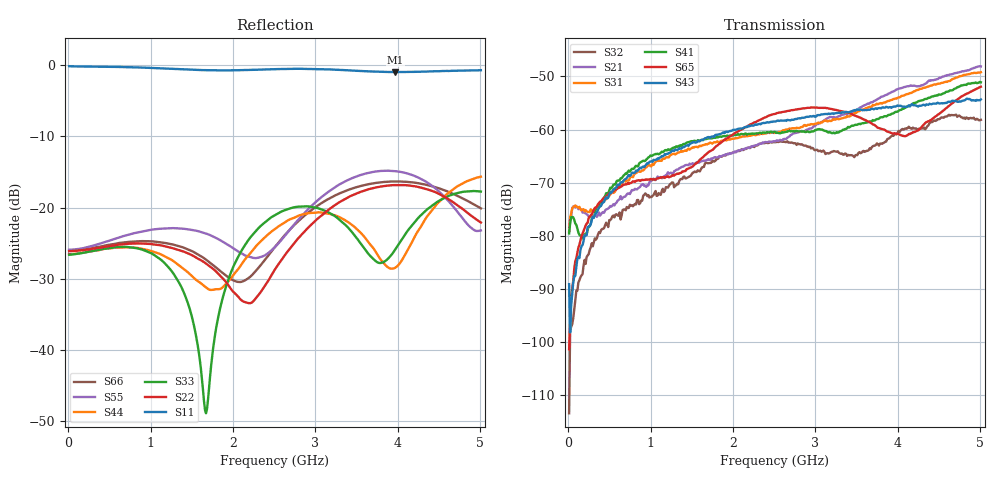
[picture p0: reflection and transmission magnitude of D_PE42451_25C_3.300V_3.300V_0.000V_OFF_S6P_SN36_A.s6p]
! Device ID: PE42451
! Serial: 36
! Insertion: A
! Temp: 25C
! VDD: 3.300
! Control_Hi: 100.000
! Control_Lo: 0.000
! Logic State: OFF
! Port 1: RFC
! Port 2: RF1
! Port 3: RF2
! Port 4: RF3
! Port 5: RF4
! Port 6: RF5
! V1 = 0.00
! V2 = 3.30
! V3 = 3.30
! V4 = 0.00
! IDD: 1.594190e-05
#  Hz  S  RI  R  50
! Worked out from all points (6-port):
!   401 points, 10 MHz to 5.01 GHz, reference 50 ohm
!   strongest paths, dB at 10 MHz, 1.26 GHz, 2.51 GHz, 3.76 GHz, 5.01 GHz:
!     S43: -89.1, -64.0, -58.5, -56.0, -54.3
!     S65: -101.4, -68.7, -57.1, -59.7, -51.9
!     S41: -79.6, -63.5, -60.4, -58.0, -51.1
!     S31: -79.1, -64.7, -60.6, -55.2, -49.2
!     S21: -79.2, -68.4, -62.3, -54.2, -48.1
!     S32: -113.5, -70.0, -62.3, -62.8, -58.2
!   lowest |S11| = -0.9 dB at 3.973 GHz (marker M1), VSWR 18.39, Z = 2.96 - j14.7 ohm
!   |S11| at or under -10 dB: nowhere
